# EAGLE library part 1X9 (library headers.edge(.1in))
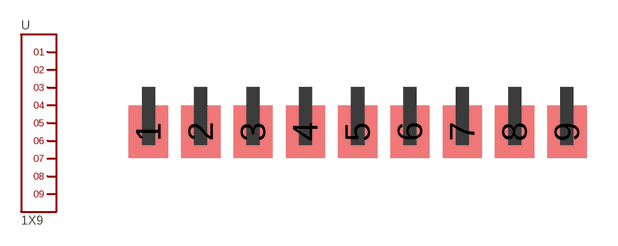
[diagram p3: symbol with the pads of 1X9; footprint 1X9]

Designator prefix -

## 1X9  [1X9]
1  1
2  2
3  3
4  4
5  5
6  6
7  7
8  8
9  9

## Footprint 1X9 (pad centres in mm)
smd 1.905 x 2.54: 1 0,-2.159; 2 2.54,-2.159; 3 5.08,-2.159; 4 7.62,-2.159; 5 10.16,-2.159; 6 12.7,-2.159; 7 15.24,-2.159; 8 17.78,-2.159; 9 20.32,-2.159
